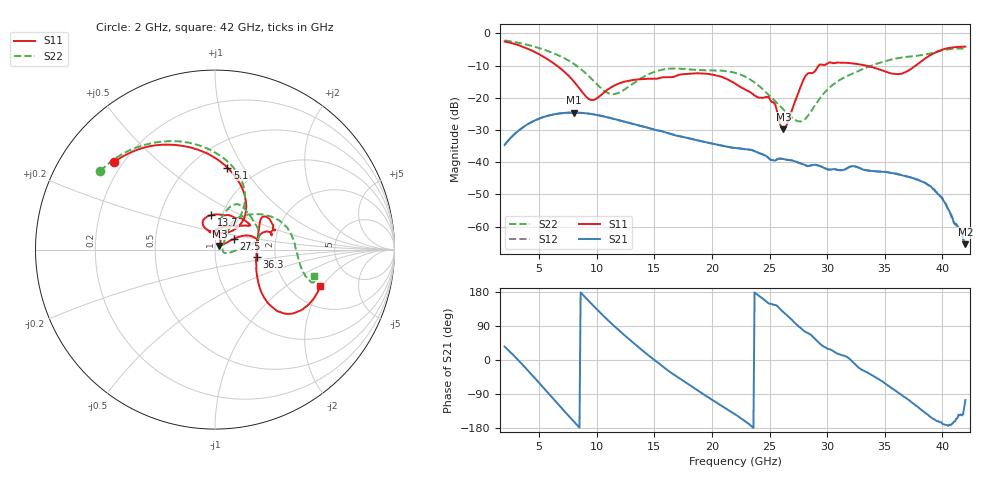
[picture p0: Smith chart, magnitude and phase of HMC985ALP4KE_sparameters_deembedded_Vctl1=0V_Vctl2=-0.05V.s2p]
!s2p File: Measurements: S11, S21, S12, S22
# GHz S dB R 50.0
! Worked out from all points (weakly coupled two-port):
!   401 points, 2 GHz to 42 GHz, reference 50 ohm
!   highest |S21| = -24.60 dB at 8 GHz (marker M1); lowest = -65.5 dB at 42 GHz (marker M2)
!   lowest |S11| = -29.8 dB at 26.2 GHz (marker M3), VSWR 1.07, Z = 52.5 + j2.2 ohm
!   |S11| at or under -10 dB: 6.526 GHz to 29.28 GHz (22.75 GHz wide, 127 % of centre); 33.34 GHz to 37.69 GHz (4.351 GHz wide, 12.3 % of centre)
!   |S22| runs from -27.4 to -2.2 dB; largest |S21 - S12| = 0.00019
!   S11 on the Smith chart (normalised r, x): 2 GHz: 0.17, +0.36; 5.1 GHz: 0.73, +0.85; 13.7 GHz: 0.89, +0.35; 27.5 GHz: 1.22, +0.15; 36.3 GHz: 1.59, -0.14; 42 GHz: 2.90, -1.91
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2  -2.55 139.3  -34.68 35.3  -34.68 35.3  -2.22 145.6
3.5  -4.06 111.4  -29.42 -10.6  -29.42 -10.6  -3.17 121.9
5.1  -6.71 81.4  -26.33 -64.0  -26.33 -64.0  -4.71 97.6
8  -14.91 44.8  -24.60 -162.1  -24.61 -162.2  -9.45 60.2
8.7  -18.09 51.5  -24.70 175.0  -24.71 175.0  -11.33 54.8
9.7  -20.70 87.4  -25.14 143.2  -25.14 143.2  -14.69 52.2
11.2  -16.88 115.8  -26.30 98.4  -26.30 98.4  -18.79 66.9
13.7  -14.29 96.7  -28.63 31.8  -28.63 31.8  -14.29 77.2
15.4  -13.94 73.0  -30.20 -9.0  -30.20 -9.0  -11.52 68.4
19.4  -12.51 34.8  -33.75 -93.1  -33.75 -93.1  -11.48 34.2
22  -15.56 52.2  -35.57 -143.1  -35.58 -143.1  -12.26 13.1
25  -20.24 97.5  -39.02 148.4  -39.02 148.4  -19.36 -4.5
26.2  -29.84 40.6  -39.03 126.2  -39.05 126.3  -23.65 -17.4
27.5  -18.43 29.5  -40.12 89.3  -40.09 89.2  -27.27 -4.6
28.1  -13.37 20.6  -40.89 74.5  -40.90 74.5  -26.57 20.3
28.7  -12.32 12.8  -40.88 63.4  -40.95 63.7  -23.70 39.6
31  -9.09 23.3  -42.44 15.6  -42.50 15.3  -14.68 57.3
33.3  -9.96 34.5  -42.43 -30.2  -42.48 -30.0  -10.84 43.1
35.4  -12.27 12.4  -43.19 -69.8  -43.24 -69.8  -8.32 26.2
36.3  -12.57 -10.1  -43.86 -89.2  -43.84 -89.2  -7.64 18.2
39.5  -5.80 -43.3  -49.23 -160.3  -49.45 -159.7  -5.73 -15.1
42  -4.14 -19.1  -65.48 -105.6  -66.07 -105.5  -4.87 -14.9
